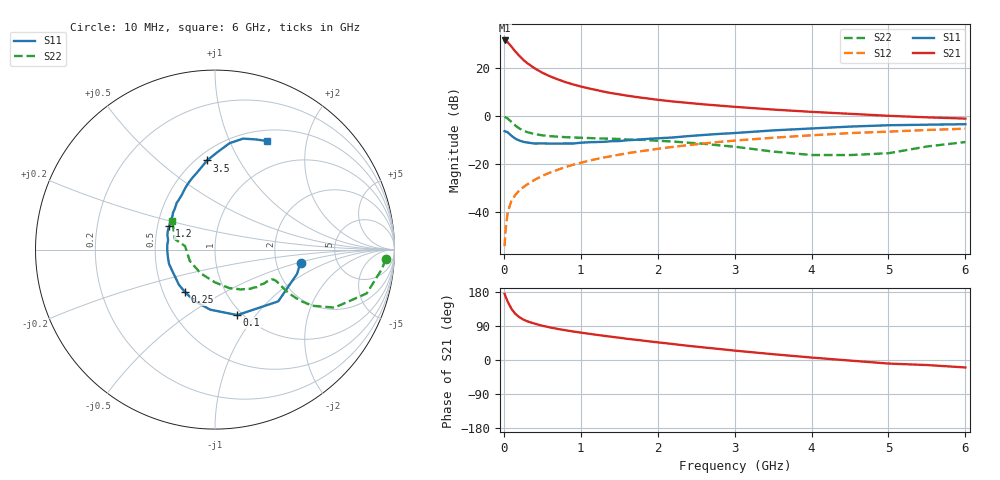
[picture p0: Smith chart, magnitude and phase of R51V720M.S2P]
! SIEMENS Small Signal Semiconductors
! BFR183
! Si NPN RF Bipolar Junction Transistor in SOT23
! VCE = 1.75 V  IC = 20 mA
! Common Emitter S-Parameters:  May  1996
# GHz  S  MA  R  50
!  f  S11  S21  S12  S22
! GHz  MAG  ANG  MAG  ANG  MAG  ANG  MAG  ANG
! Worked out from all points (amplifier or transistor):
!   36 points, 10 MHz to 6 GHz, reference 50 ohm
!   highest |S21| = 31.2 dB at 10 MHz (marker M1)
!   |S21| within 3 dB of that: start of sweep to 110.6 MHz
!   unconditionally stable (mu >= 1): 503.9 MHz to 2.398 GHz
!   at 250 MHz: K = 0.83, MSG = 26.4 dB, |S12| = -29.6 dB
!   at 1.4 GHz: K = 1.06, MAG = 11.6 dB, |S12| = -16.7 dB
!   at 6 GHz: K = 0.91, MSG = 2.1 dB, |S12| = -5.3 dB
!   S11 on the Smith chart (normalised r, x): 10 MHz: 2.75, -0.52; 100 MHz: 0.95, -0.81; 250 MHz: 0.65, -0.33; 1.2 GHz: 0.58, +0.16; 3.5 GHz: 0.56, +0.74; 6 GHz: 0.63, +1.38
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0.01  0.4819 -8.6  36.3 174.4  0.002 91.2  0.9535 -3.2
0.02  0.4767 -16.5  36 168.7  0.004 84.2  0.9349 -6.8
0.05  0.4552 -39.3  33.36 153.9  0.0101 76.1  0.8798 -16.1
0.1  0.3853 -71.2  26.98 134.8  0.0178 68.9  0.7402 -25.9
0.15  0.336 -94.4  21.43 121.7  0.0231 66.8  0.6258 -30.0
0.2  0.3087 -111.5  17.51 113.3  0.0284 67.2  0.55 -31.0
0.25  0.2898 -125.2  14.57 107.0  0.033 67.1  0.4962 -30.7
0.3  0.2808 -135.7  12.45 102.4  0.0376 68.6  0.4615 -30.2
0.4  0.2666 -150.7  9.646 96.0  0.0472 69.9  0.4192 -28.7
0.5  0.2683 -162.8  7.794 90.4  0.0571 70.8  0.3938 -27.6
0.6  0.2657 -172.1  6.569 86.0  0.0668 71.0  0.3793 -27.1
0.7  0.266 -179.6  5.686 82.0  0.0763 71.1  0.3697 -27.1
0.8  0.2671 174.5  4.987 78.5  0.0866 70.7  0.361 -27.4
0.9  0.2669 168.3  4.465 75.3  0.0969 69.8  0.3554 -27.8
1.1  0.2833 158.0  3.71 69.5  0.1169 68.9  0.3469 -30.0
1.2  0.2862 153.0  3.424 66.6  0.1271 68.1  0.3416 -31.0
1.6  0.3115 138.7  2.614 56.1  0.1671 64.2  0.3237 -36.7
2.2  0.3565 121.2  1.977 42.1  0.2275 57.7  0.2935 -48.0
3.5  0.4986 95.1  1.347 15.3  0.3515 40.8  0.1818 -90.5
4.5  0.5982 82.2  1.1 -1.5  0.4388 27.7  0.1539 -155.7
5.5  0.6545 69.7  0.93 -13.3  0.5087 15.7  0.2314 165.3
6  0.6701 64.6  0.875 -19.7  0.541 8.0  0.2863 146.1
